(* Logix 5000 AddOnInstructionDefinition export AMCI_3202_AOP_Absolute_Move; software revision 20.03 *)

ADD_ON_INSTRUCTION AMCI_3202_AOP_Absolute_Move   (* revision 1.0, vendor AMCI, ExecuteEnableInFalse *)
VAR_INPUT
   axis_status_bits : INT; {required}
   channel_number : INT; {required}
   _0_normal_1_S_Curve_Acceleration : BOOL;
   _0_Triangular_1_Trapezoidal_S_Curve : BOOL;
   _0_Target_Position_1_Encoder_Move : BOOL;
   Target_Position : DINT; {required}
   Programmed_speed : DINT; {required}
   Acceleration : DINT; {required}
   Deceleration : DINT; {required}
END_VAR
VAR_IN_OUT
   AMCI_3202_output_data : AM:1756_3202:O:0; {required}
END_VAR
VAR_OUTPUT
   EN : BOOL; {access Read Only, visible}
   ER : BOOL; {access Read Only, visible}
END_VAR
VAR
   command_data_block : DINT[8]; {access None}
END_VAR

ROUTINE EnableInFalse   (* ladder *)
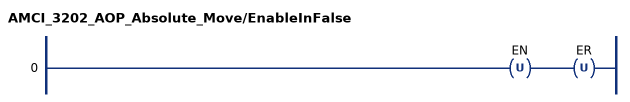
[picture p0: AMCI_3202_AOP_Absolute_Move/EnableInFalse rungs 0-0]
   0: OTU(EN)OTU(ER);
END_ROUTINE

ROUTINE Logic   (* ladder *)
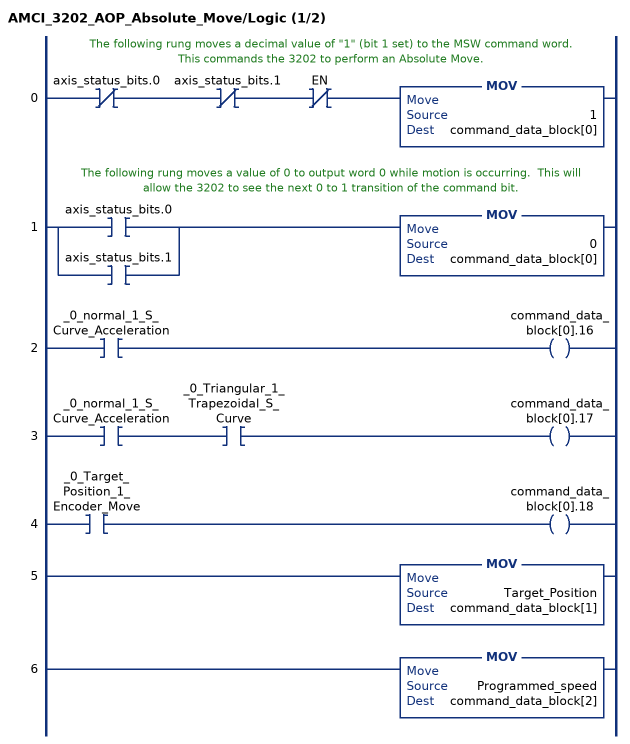
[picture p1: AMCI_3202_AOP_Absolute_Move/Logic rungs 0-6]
   // The following rung moves a decimal value of "1" (bit 1 set) to the MSW command word.  This commands the 3202 to perform an Absolute Move.
   0: XIO(axis_status_bits.0)XIO(axis_status_bits.1)XIO(EN)MOV(1,command_data_block[0]);
   // The following rung moves a value of 0 to output word 0 while motion is occurring.  This will allow the 3202 to see the next 0 to 1 transition of the command bit.
   1: [XIC(axis_status_bits.0) ,XIC(axis_status_bits.1) ]MOV(0,command_data_block[0]);
   2: XIC(_0_normal_1_S_Curve_Acceleration)OTE(command_data_block[0].16);
   3: XIC(_0_normal_1_S_Curve_Acceleration)XIC(_0_Triangular_1_Trapezoidal_S_Curve)OTE(command_data_block[0].17);
   4: XIC(_0_Target_Position_1_Encoder_Move)OTE(command_data_block[0].18);
   5: MOV(Target_Position,command_data_block[1]);
   6: MOV(Programmed_speed,command_data_block[2]);
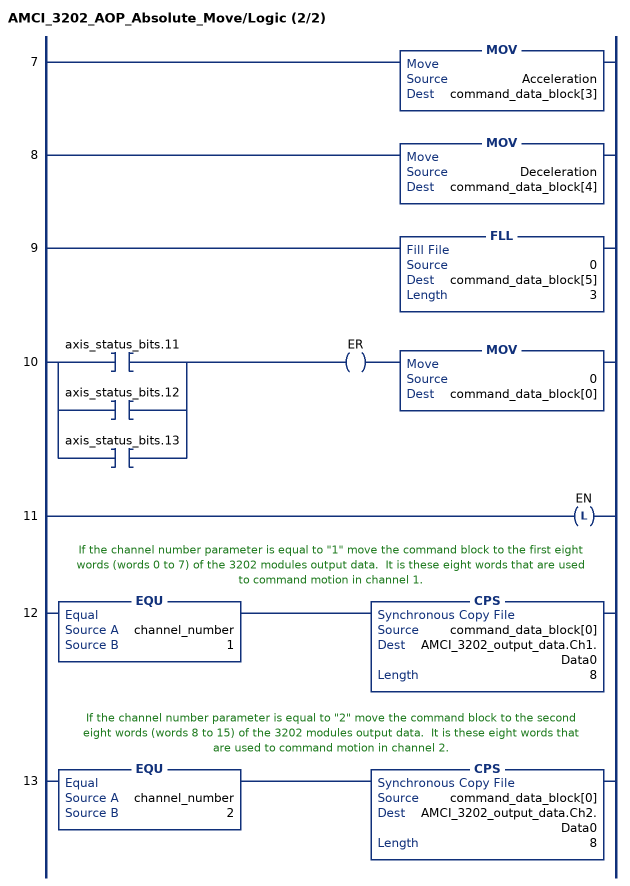
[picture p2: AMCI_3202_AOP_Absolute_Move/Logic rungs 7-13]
   7: MOV(Acceleration,command_data_block[3]);
   8: MOV(Deceleration,command_data_block[4]);
   9: FLL(0,command_data_block[5],3);
   10: [XIC(axis_status_bits.11) ,XIC(axis_status_bits.12) ,XIC(axis_status_bits.13) ]OTE(ER)MOV(0,command_data_block[0]);
   11: OTL(EN);
   // If the channel number parameter is equal to "1" move the command block to the first eight words (words 0 to 7) of the 3202 modules output data.  It is these eight words that are used to command motion in channel 1.
   12: EQU(channel_number,1)CPS(command_data_block[0],AMCI_3202_output_data.Ch1.Data0,8);
   // If the channel number parameter is equal to "2" move the command block to the second eight words (words 8 to 15) of the 3202 modules output data.  It is these eight words that are used to command motion in channel 2.
   13: EQU(channel_number,2)CPS(command_data_block[0],AMCI_3202_output_data.Ch2.Data0,8);
END_ROUTINE
END_ADD_ON_INSTRUCTION
